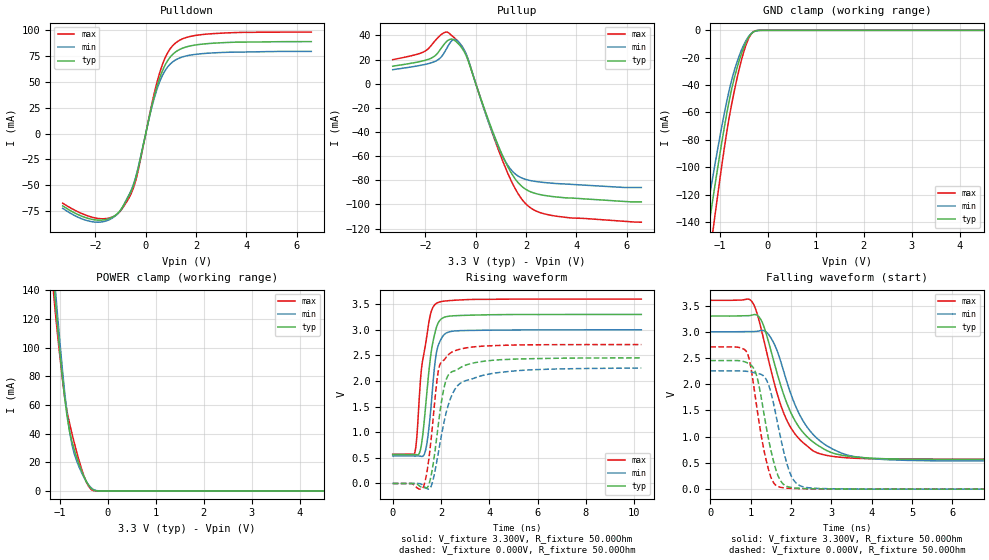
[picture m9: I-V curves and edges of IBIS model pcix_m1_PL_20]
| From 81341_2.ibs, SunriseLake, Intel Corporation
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[Model]   pcix_m1_PL_20
Model_type   I/O
Vinl = 1.155V
Vinh = 1.650V
Vmeas = 1.320V
Vref = 0.000V
Cref = 10.000pF
Rref = 25.000Ohm
|   typ   min   max
C_comp   7.500pF   6.000pF   9.000pF
[Voltage Range]   3.300V   3.000V   3.600V
[Temperature Range]   60.0   110.0   -5.0
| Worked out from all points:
|   slope of the pulldown table from 0 to 0.495 V, typ, clamps not added: 9.98 ohm
|   slope of the pullup table from 0 to 0.495 V, typ, clamps not added: 16.6 ohm
|   GND clamp passes 1 mA (typ) near -0.30 V on its own axis
|   POWER clamp passes 1 mA (typ) near -0.32 V on its own axis
|   falling waveform, V_fixture 3.300V, R_fixture 50.00Ohm: 20-80 % time 805ps typ, 849ps min, 711ps max; typ from 3.3 V to 0.565 V
|   rising waveform, V_fixture 3.300V, R_fixture 50.00Ohm: 20-80 % time 379ps typ, 309ps min, 411ps max; typ from 0.565 V to 3.3 V
|   rising waveform, V_fixture 0.000V, R_fixture 50.00Ohm: 20-80 % time 464ps typ, 700ps min, 367ps max; typ from 0 V to 2.45 V
|   falling waveform, V_fixture 0.000V, R_fixture 50.00Ohm: 20-80 % time 372ps typ, 398ps min, 350ps max; typ from 2.45 V to 0 V
[Pulldown]
|   Voltage   I(typ)   I(min)   I(max)
-3.3V     -70.16mA   -72.52mA   -67.63mA
-1.9V     -83.98mA   -85.97mA   -82.3mA
-1.35V    -81.34mA   -82.29mA   -81.19mA
-950mV    -72.25mA   -72.54mA   -73.2mA
-600mV    -56.91mA   -56.02mA   -59.24mA
-400mV    -43.19mA   -42.17mA   -45.6mA
200mV     22.51mA    21.68mA    24.14mA
500mV     49.98mA    46.89mA    54.63mA
850mV     70.01mA    64.03mA    77.52mA
1.25V     80.23mA    72.29mA    89.06mA
2.65V     87.59mA    78.2mA     96.89mA
6.575V    89.19mA    79.71mA    98.42mA
[GND Clamp]
|   Voltage   I(typ)   I(min)   I(max)
-3.3V     -632.5mA   -564.4mA   -725.5mA
-1.325V   -165.6mA   -144.4mA   -196mA
-1.3V     -159.5mA   -139mA     -189mA
-1.25V    -147.6mA   -128.4mA   -175.3mA
-1.2V     -135.8mA   -118mA     -161.6mA
-1.125V   -118.5mA   -102.6mA   -141.4mA
-850mV    -59.64mA   -50.8mA    -72.97mA
-650mV    -28.41mA   -23.93mA   -36.31mA
-450mV    -8.219mA   -7.112mA   -10.14mA
-350mV    -2.584mA   -2.413mA   -2.802mA
-250mV    -331.3uA   -398.2uA   -220.5uA
6.575V    0A         0A         0A
[Pullup]
|   Voltage   I(typ)   I(min)   I(max)
-3.3V     14.46mA    11.58mA    19.88mA
-1.8V     20.83mA    17.09mA    30.91mA
-1.4V     28.55mA    21.52mA    40.19mA
-1.1V     35.94mA    31.22mA    42.38mA
-850mV    35.95mA    36.64mA    37.96mA
-500mV    27.86mA    29.38mA    29.24mA
500mV     -30.03mA   -31.44mA   -31.45mA
1V        -56.62mA   -57.35mA   -60.36mA
1.5V      -76.94mA   -73.54mA   -84.4mA
2V        -87.7mA    -79.4mA    -99.81mA
3.2V      -93.84mA   -82.73mA   -109.7mA
6.575V    -97.91mA   -86.02mA   -114.7mA
[POWER Clamp]
|   Voltage   I(typ)   I(min)   I(max)
-3.3V     1.109A     1.089A     1.13A
-1.15V    154.7mA    163.7mA    144.9mA
-1.1V     134.6mA    143.1mA    126.4mA
-1.05V    115.4mA    123.1mA    109.5mA
-900mV    64.86mA    68.99mA    65.55mA
-800mV    41.99mA    41.86mA    47.4mA
-750mV    34.63mA    32.54mA    40.32mA
-650mV    23.51mA    20.95mA    27.23mA
-500mV    10.16mA    9.585mA    10.63mA
-400mV    3.792mA    4.116mA    3.102mA
-300mV    590.1uA    959uA      205.5uA
6.575V    0A         0A         0A
[Ramp]
R_load = 50.00Ohm
|   typ   min   max
dV/dt_r   1.471V/463.461ps   1.352V/699.345ps   1.627V/366.358ps
dV/dt_f   1.641V/804.337ps   1.478V/849.154ps   1.816V/710.731ps
[Falling Waveform]
V_fixture = 3.300V
V_fixture_min = 3.000V
V_fixture_max = 3.600V
R_fixture = 50.00Ohm
|   Time   V(typ)   V(min)   V(max)
0s        3.3V       3V         3.6V
1.04ns    3.319V     3.005V     3.568V
1.24ns    3.249V     3.022V     3.123V
1.45ns    2.792V     2.944V     2.442V
1.85ns    1.739V     2.168V     1.396V
2.23ns    1.151V     1.397V     938.2mV
2.65ns    844.3mV    966.2mV    692.6mV
3.24ns    650.6mV    691.7mV    607.3mV
3.96ns    592.1mV    582.9mV    580.5mV
10.3ns    565.2mV    536.6mV    572.6mV
[Rising Waveform]
V_fixture = 3.300V
V_fixture_min = 3.000V
V_fixture_max = 3.600V
R_fixture = 50.00Ohm
|   Time   V(typ)   V(min)   V(max)
0s        565.2mV    536.6mV    572.6mV
910ps     565.3mV    536.1mV    595.5mV
1ns       560.6mV    536.4mV    913mV
1.12ns    609.1mV    534.5mV    1.812V
1.21ns    821mV      528.4mV    2.31V
1.42ns    1.798V     794.6mV    2.899V
1.6ns     2.58V      1.565V     3.361V
1.82ns    3.059V     2.573V     3.519V
2.48ns    3.272V     2.973V     3.574V
10.3ns    3.3V       3V         3.6V
[Rising Waveform]
V_fixture = 0.000V
V_fixture_min = 0.000V
V_fixture_max = 0.000V
R_fixture = 50.00Ohm
|   Time   V(typ)   V(min)   V(max)
0s        559.7nV    3.313uV    41.29nV
1.27ns    -79.43mV   -46.65mV   -67.86mV
1.41ns    -85.09mV   -97.65mV   201.6mV
1.56ns    84.56mV    -85.15mV   729.7mV
1.91ns    1.221V     651.2mV    2.244V
2.16ns    1.936V     1.273V     2.429V
2.44ns    2.177V     1.711V     2.561V
2.92ns    2.291V     1.988V     2.636V
4.29ns    2.411V     2.159V     2.693V
10.3ns    2.452V     2.254V     2.711V
[Falling Waveform]
V_fixture = 0.000V
V_fixture_min = 0.000V
V_fixture_max = 0.000V
R_fixture = 50.00Ohm
|   Time   V(typ)   V(min)   V(max)
0s        2.452V     2.254V     2.711V
910ps     2.41V      2.245V     2.603V
1.01ns    2.362V     2.234V     2.304V
1.14ns    2.186V     2.21V      1.635V
1.39ns    1.177V     2.085V     538.5mV
1.54ns    619.5mV    1.728V     162.4mV
1.7ns     220.4mV    1.14V      44.04mV
2ns       32.02mV    264.4mV    14.95mV
2.37ns    11.77mV    33.44mV    6.23mV
10.3ns    559.7nV    3.313uV    41.29nV
